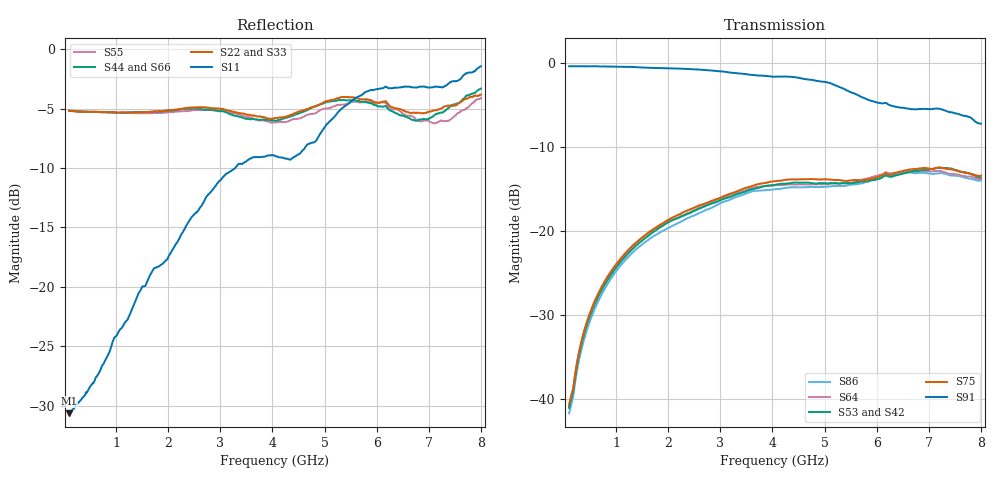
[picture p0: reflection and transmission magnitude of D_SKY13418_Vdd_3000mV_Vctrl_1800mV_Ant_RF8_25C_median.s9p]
# GHz S DB R 50
! THRU S21 mag phase subtraction.
! HALF_THRU
! EN33-165-011-v1_HALF_THRU_1 EN33-165-011-v1_HALF_THRU_2 EN33-165-011-v1_HALF_THRU_3 EN33-165-011-v1_HALF_THRU_4 EN33-165-011-v1_HALF_THRU_5 EN33-165-011-v1_HALF_THRU_6 EN33-165-011-v1_HALF_THRU_7 EN33-165-011-v1_HALF_THRU_8 EN33-165-011-v1_HALF_THRU_9
! THRU Ports: 1 2
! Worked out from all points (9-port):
!   801 points, 100 MHz to 8 GHz, reference 50 ohm
!   strongest paths, dB at 100 MHz, 2.075 GHz, 4.05 GHz, 6.025 GHz, 8 GHz:
!     S91: -0.4, -0.7, -1.6, -4.7, -7.2
!     S75: -40.6, -18.4, -14.1, -13.5, -13.4
!     S53: -41.0, -18.7, -14.5, -13.8, -13.6
!     S64: -40.8, -18.7, -14.5, -13.4, -13.8
!     S42: -41.0, -18.9, -14.7, -13.5, -13.6
!     S86: -41.7, -19.4, -15.0, -13.7, -14.0
!   lowest |S11| = -30.6 dB at 100 MHz (marker M1), VSWR 1.06, Z = 53 + j0.0429 ohm
!   |S11| at or under -10 dB: start of sweep to 3.287 GHz
